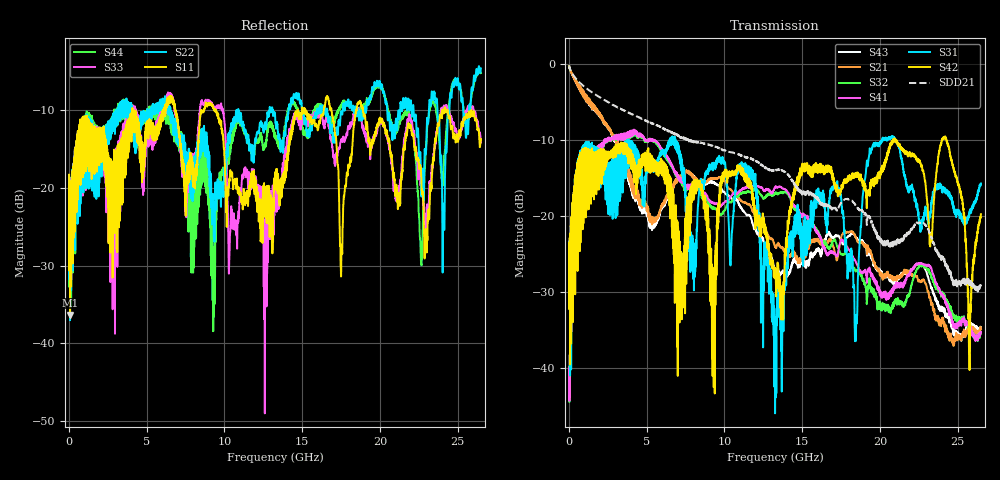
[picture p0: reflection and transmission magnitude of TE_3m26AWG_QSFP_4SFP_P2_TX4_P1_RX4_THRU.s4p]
!Agilent Technologies,N5222A,MY51421691,A.10.00.00
!Agilent N5222A: A.10.00.00
!Date: Friday, January 30, 2015 12:33:43
!Correction: S11(Full 4 Port(1,2,3,4))
!S12(Full 4 Port(1,2,3,4))
!S13(Full 4 Port(1,2,3,4))
!S14(Full 4 Port(1,2,3,4))
!S21(Full 4 Port(1,2,3,4))
!S22(Full 4 Port(1,2,3,4))
!S23(Full 4 Port(1,2,3,4))
!S24(Full 4 Port(1,2,3,4))
!S31(Full 4 Port(1,2,3,4))
!S32(Full 4 Port(1,2,3,4))
!S33(Full 4 Port(1,2,3,4))
!S34(Full 4 Port(1,2,3,4))
!S41(Full 4 Port(1,2,3,4))
!S42(Full 4 Port(1,2,3,4))
!S43(Full 4 Port(1,2,3,4))
!S44(Full 4 Port(1,2,3,4))
!S4P File: Measurements: <S11,S12,S13,S14>,
!<S21,S22,S23,S24>,
!<S31,S32,S33,S34>,
!<S41,S42,S43,S44>:
# Hz S  dB  R 50.0
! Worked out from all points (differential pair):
!   2650 points, 10 MHz to 26.5 GHz, reference 50 ohm
!   strongest paths, dB at 10 MHz, 6.63 GHz, 13.26 GHz, 19.88 GHz, 26.5 GHz:
!     S42: -25.1, -19.6, -27.0, -15.0, -19.8
!     S31: -25.1, -10.5, -45.9, -10.4, -15.7
!     S41: -40.1, -13.4, -16.3, -29.7, -35.3
!     S32: -40.6, -13.6, -17.1, -32.1, -35.2
!     S21: -0.4, -16.5, -24.1, -27.2, -34.9
!     S43: -0.3, -16.7, -27.6, -27.3, -34.7
!   taken as a pair (ports 1,3 in; 2,4 out), SDD21 dB: -0.3, -9.1, -14.1, -23.0, -29.1
!   lowest |S11| = -36.4 dB at 70 MHz (marker M1), VSWR 1.03, Z = 51.4 + j0.732 ohm
!   |S11| at or under -10 dB: start of sweep to 4.075 GHz; 9.454 GHz to 14.73 GHz (5.275 GHz wide, 43.6 % of centre); 18.91 GHz to 24.01 GHz (5.102 GHz wide, 23.8 % of centre)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
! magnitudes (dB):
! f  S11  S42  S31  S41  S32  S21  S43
! 10 MHz  -18.3  -25.1  -25.1  -40.1  -40.6  -0.4  -0.3
! 70 MHz  -36.4  -39.5  -41.0  -40.9  -41.1  -0.8  -0.8
! 4.19 GHz  -10.0  -12.6  -10.7  -9.3  -9.4  -16.4  -16.6
! 9.28 GHz  -9.8  -39.0  -13.1  -18.3  -18.9  -15.1  -15.6
! 13.25 GHz  -19.4  -27.9  -36.7  -16.3  -17.0  -24.1  -27.6
! 22.65 GHz  -18.1  -13.4  -21.9  -26.2  -26.6  -28.5  -26.4
! 26.5 GHz  -13.8  -19.8  -15.7  -35.3  -35.2  -34.9  -34.7
